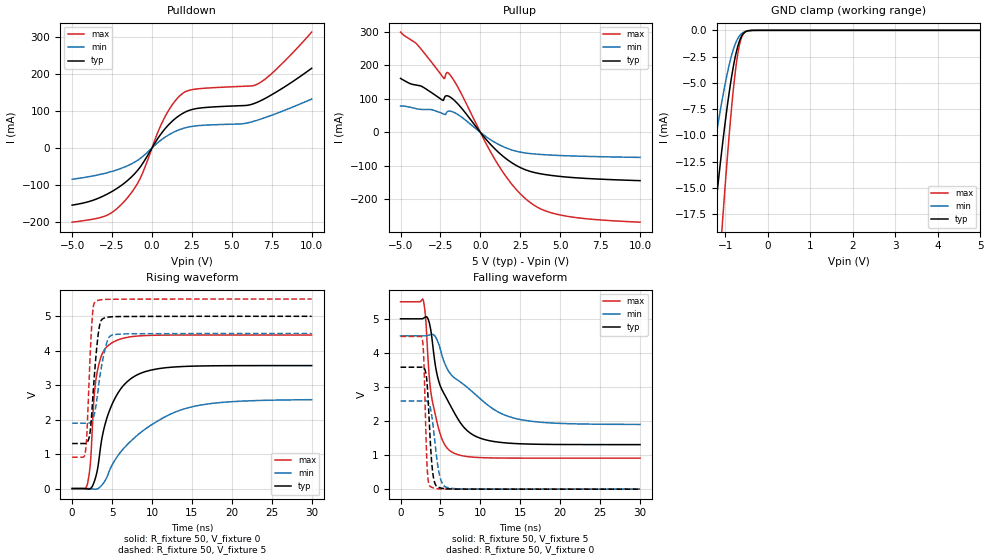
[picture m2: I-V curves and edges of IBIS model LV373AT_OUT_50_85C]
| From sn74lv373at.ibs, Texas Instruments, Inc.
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[Model]   LV373AT_OUT_50_85C
Model_type  3-state
Enable   Active-Low
Vref =   0
Rref =   1000
Cref =   50p
Vmeas =   1.5
| variable   typ   min   max
C_comp   4.52pF   3.43pF   5.27pF
| C_pullup   7.24pF   3.72pF   11.86pF
| C_pulldown   7.11pF   4.35pF   11.55pF
| C_tri-state   4.52pF   3.43pF   5.27pF
[Temperature Range]   40   100   -40
| Ambient temperature   25   85   -40
[Voltage range]   5   4.5   5.5
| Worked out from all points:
|   slope of the pulldown table from 0 to 0.75 V, typ, clamps not added: 15.5 ohm
|   slope of the pullup table from 0 to 0.75 V, typ, clamps not added: 18 ohm
|   GND clamp passes 1 mA (typ) near -0.67 V on its own axis
|   rising waveform, R_fixture 50, V_fixture 0: 20-80 % time 2.69ns typ, 6.81ns min, 968ps max; typ from 0 V to 3.57 V
|   falling waveform, R_fixture 50, V_fixture 5: 20-80 % time 3.21ns typ, 6.07ns min, 1.45ns max; typ from 5 V to 1.31 V
|   rising waveform, R_fixture 50, V_fixture 5: 20-80 % time 740ps typ, 1.06ns min, 517ps max; typ from 1.31 V to 5 V
|   falling waveform, R_fixture 50, V_fixture 0: 20-80 % time 533ps typ, 827ps min, 336ps max; typ from 3.58 V to 0 V
[GND Clamp]
| LV373AT_OUT_50
|   Voltage   I(typ)   I(min)   I(max)
-5V       -241.3mA   -158mA     -307.6mA
-1.56V    -30.91mA   -19.51mA   -48.95mA
-1.51V    -28.62mA   -18.02mA   -45.62mA
-1.28V    -18.74mA   -11.59mA   -30.78mA
-1.08V    -11.23mA   -6.683mA   -18.84mA
-1.06V    -10.54mA   -6.237mA   -17.72mA
-885mV    -5.19mA    -2.847mA   -8.691mA
-775mV    -2.635mA   -1.364mA   -4.197mA
-675mV    -1.074mA   -559.6uA   -1.486mA
-625mV    -591.6uA   -329.6uA   -730.9uA
-555mV    -210.9uA   -140.8uA   -215.4uA
5V        79.3nA     5.28nA     758.3nA
[Pulldown]
| LV373AT_OUT_50
|   Voltage   I(typ)   I(min)   I(max)
-5V       -154.5mA   -84.56mA   -200.6mA
-2.855V   -125.8mA   -67.44mA   -182.5mA
-1.595V   -90.3mA    -49.23mA   -137.6mA
-700mV    -49.38mA   -27.23mA   -78.76mA
325mV     23.07mA    12.87mA    38.05mA
815mV     51.71mA    28.99mA    84.22mA
1.34V     75.09mA    42.2mA     120.9mA
1.87V     91.96mA    51.64mA    145.8mA
2.85V     107mA      60.16mA    159.7mA
6.575V    123.1mA    74.71mA    172mA
7.735V    149.9mA    92.26mA    210.6mA
10V       215.3mA    132.1mA    313.1mA
[Pullup]
| LV373AT_OUT_50
|   Voltage   I(typ)   I(min)   I(max)
-5V       160.9mA    78.57mA    299.3mA
-3.98V    140.8mA    70.18mA    263.3mA
-3.065V   118.7mA    67.93mA    209.8mA
-2.285V   99.16mA    54.49mA    161.1mA
-2.09V    109.1mA    60.99mA    178.5mA
-1.855V   104.2mA    62.95mA    169mA
1.08V     -57.26mA   -34.59mA   -94.33mA
2.055V    -93.47mA   -53.89mA   -159.9mA
3.015V    -115mA     -62.85mA   -205.7mA
3.945V    -125.2mA   -66.56mA   -232.1mA
5.19V     -132.6mA   -69.59mA   -248.6mA
10V       -144.3mA   -74.87mA   -268.3mA
[Ramp]
| LV373AT_OUT_50
| variable   typ   min   max
dV/dt_r   2.15/2.69E-09   1.56/6.81E-09   2.67/9.64E-10
dV/dt_f   2.25/3.20E-09   1.59/6.06E-09   2.80/1.45E-09
R_load = 50
[Rising Waveform]
| LV373AT_OUT_50
R_fixture =   50
C_fixture =   0
L_fixture =   0
V_fixture =   0
V_fixture_min = 0
V_fixture_max = 0
|   Time   V(typ)   V(min)   V(max)
0s        1.266nV    819pV      2.497nV
1.9ns     -11mV      490.5uV    120.7mV
2.285ns   409.9uV    -4.108mV   733.8mV
2.71ns    162.6mV    -14.69mV   2.537V
3.085ns   456.2mV    -13.34mV   3.314V
3.9ns     1.651V     150.1mV    3.975V
4.94ns    2.413V     655.8mV    4.223V
7.915ns   3.273V     1.497V     4.421V
13.69ns   3.541V     2.288V     4.456V
29.99ns   3.569V     2.579V     4.457V
[Falling Waveform]
| LV373AT_OUT_50
R_fixture =   50
C_fixture =   0
L_fixture =   0
V_fixture =   5
V_fixture_min = 4.5
V_fixture_max = 5.5
|   Time   V(typ)   V(min)   V(max)
0s        5V         4.5V       5.5V
2.83ns    5.01V      4.499V     5.561V
3.145ns   5.054V     4.501V     5.024V
3.43ns    5.004V     4.515V     3.87V
3.95ns    4.398V     4.546V     2.628V
4.77ns    3.181V     4.266V     1.778V
6.34ns    2.414V     3.359V     1.102V
9.075ns   1.593V     2.843V     939.6mV
14.2ns    1.341V     2.086V     911.5mV
29.99ns   1.308V     1.9V       910.3mV
[Rising Waveform]
| LV373AT_OUT_50
R_fixture =   50
C_fixture =   0
L_fixture =   0
V_fixture =   5
V_fixture_min = 4.5
V_fixture_max = 5.5
|   Time   V(typ)   V(min)   V(max)
0s        1.308V     1.898V     910.3mV
1.665ns   1.309V     1.898V     1.067V
1.85ns    1.332V     1.896V     1.595V
2.17ns    1.527V     1.905V     3.388V
2.49ns    2.286V     1.976V     4.862V
2.98ns    3.835V     2.399V     5.438V
3.58ns    4.853V     3.415V     5.479V
4.345ns   4.97V      4.239V     5.492V
4.97ns    4.985V     4.45V      5.494V
29.99ns   5V         4.5V       5.5V
[Falling Waveform]
| LV373AT_OUT_50
R_fixture =   50
C_fixture =   0
L_fixture =   0
V_fixture =   0
V_fixture_min = 0
V_fixture_max = 0
|   Time   V(typ)   V(min)   V(max)
0s        3.579V     2.588V     4.481V
2.735ns   3.583V     2.589V     4.389V
2.92ns    3.569V     2.591V     3.78V
3.34ns    3.063V     2.58V      616.9mV
3.75ns    1.319V     2.362V     72.66mV
4ns       556.3mV    2.005V     45.43mV
4.3ns     175.1mV    1.398V     24.58mV
4.905ns   43.45mV    391.5mV    8.306mV
5.695ns   12.87mV    60.68mV    3.1mV
29.99ns   289.3nV    4.823uV    8.501nV
